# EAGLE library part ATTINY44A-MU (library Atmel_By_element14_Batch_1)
Microcontroller with In-System Programmable Flash
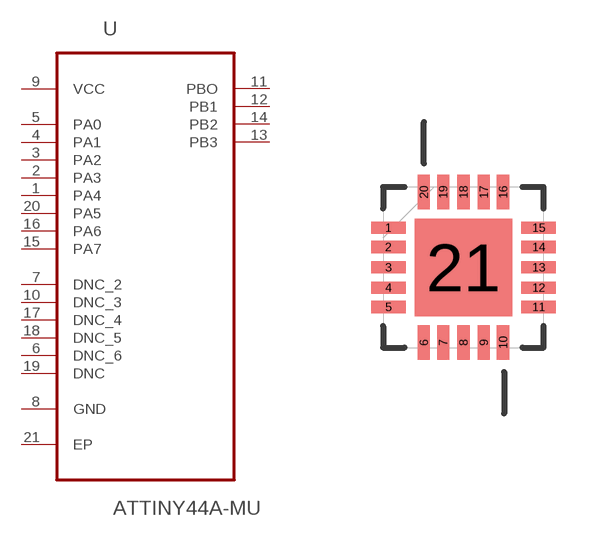
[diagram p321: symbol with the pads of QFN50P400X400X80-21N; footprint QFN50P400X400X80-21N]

Designator prefix U

## ATTINY44A-MU (MPN: ATTINY44A-MU; OC_FARNELL: 1748545; OC_NEWARK: 26R5651; PACKAGE: QFN-20; SUPPLIER: Atmel)  [QFN50P400X400X80-21N]
1  PA4
2  PA3
3  PA2
4  PA1
5  PA0
6  DNC_6  nc
7  DNC_2  nc
8  GND  pas
9  VCC  pwr
10  DNC_3  nc
11  PBO
12  PB1
13  PB3
14  PB2
15  PA7
16  PA6
17  DNC_4  nc
18  DNC_5  nc
19  DNC  nc
20  PA5
21  EP  pas

## Footprint QFN50P400X400X80-21N (pad centres in mm)
smd 0.864 x 0.305: 1 -1.88,0.991; 2 -1.88,0.508; 3 -1.88,0; 4 -1.88,-0.508; 5 -1.88,-0.991; 11 1.88,-0.991; 12 1.88,-0.508; 13 1.88,0; 14 1.88,0.508; 15 1.88,0.991
smd 0.305 x 0.864: 6 -0.991,-1.88; 7 -0.508,-1.88; 8 0,-1.88; 9 0.508,-1.88; 10 0.991,-1.88; 16 0.991,1.88; 17 0.508,1.88; 18 0,1.88; 19 -0.508,1.88; 20 -0.991,1.88
smd 2.438 x 2.438: 21 0,0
